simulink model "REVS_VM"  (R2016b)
settings: Solver=ode3  StartTime=REVS.sim_start_time_secs  StopTime=Inf  FixedStep=REVS.sim_step_time_secs  MaxStep=REVS.sim_step_time_secs  EnableMultiTasking=on
StopFcn:
  | postproc_datalog;
  | postproc_audit;
  | postproc_result;
model workspace (MATLAB code in the model file):
  other statements: REVS_setup_variants
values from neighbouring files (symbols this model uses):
  accessory = class_accessory_data    [class_test_data.m]
  battery = class_battery_data    [class_accessory_data.m]    (also in class_REVS_electric.m = class_REVS_battery)
  brake = struct(	'max_torque_Nm',[], 						'proportion_norm',1.0, 						'inertia_kgm2',0.0)    [class_REVS_drive_axle.m]
  engine = class_engine_data    [class_test_data.m]
  final_drive = struct(	'gear_ratio',[], 								'efficiency_norm',[], 								'inertia_kgm2',[] )    [class_REVS_drive_axle.m]
  gear = class_REVS_gearbox    [class_REVS_AT_transmission.m]
  tire = struct(	'radius_m',[], 						'rolling_resistance_coefficient',0, 						'vehicle_weight_norm',1.0,  						'wheel_slip_torque_Nm',[],  						'inertia_kgm2',0.0)    [class_REVS_drive_axle.m]
  torque_converter = class_REVS_torque_converter    [class_REVS_AT_transmission.m]
  transmission = class_transmission_data    [class_test_data.m]
  vehicle = class_vehicle_data    [class_test_data.m]
undefined symbols (not defined in the file or in its folder): alternator, ambient, controls, convert, DelayTimeSecs, drive_cycle, driver, electric, gear_strategy, InitialCondition, InitialValue, LoadSource, LookupStructure, MultiplyPosInputs, Normalize, NumPhases, REVS, SpeedSource, starter, tableshift, UpperSaturationLimit, Value, VerboseLevel, VerboseSignal
libraries: simulink x153
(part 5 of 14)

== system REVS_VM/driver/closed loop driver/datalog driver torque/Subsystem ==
  In1 : Inport
  Enable : EnablePort
  To Workspace : ToWorkspace  VariableName=datalog__driver__p_pedal_unscaled  SampleTime=-1
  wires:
  In1/1 -> To Workspace/1

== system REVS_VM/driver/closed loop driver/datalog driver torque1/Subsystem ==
  In1 : Inport
  Enable : EnablePort
  To Workspace : ToWorkspace  VariableName=datalog__driver__i_pedal_unscaled  SampleTime=-1
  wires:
  In1/1 -> To Workspace/1

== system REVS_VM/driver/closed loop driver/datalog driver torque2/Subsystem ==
  In1 : Inport
  Enable : EnablePort
  To Workspace : ToWorkspace  VariableName=datalog__driver__d_pedal_unscaled  SampleTime=-1
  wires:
  In1/1 -> To Workspace/1

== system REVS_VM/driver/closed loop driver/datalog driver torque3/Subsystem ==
  In1 : Inport
  Enable : EnablePort
  To Workspace : ToWorkspace  VariableName=datalog__driver__driveline_enagaged_bool  SampleTime=-1
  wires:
  In1/1 -> To Workspace/1

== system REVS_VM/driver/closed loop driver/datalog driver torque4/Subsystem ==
  In1 : Inport
  Enable : EnablePort
  To Workspace : ToWorkspace  VariableName=datalog__driver__driveline_enagaged_norm  SampleTime=-1
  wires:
  In1/1 -> To Workspace/1

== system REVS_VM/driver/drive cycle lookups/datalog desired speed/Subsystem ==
  In1 : Inport
  Enable : EnablePort
  To Workspace : ToWorkspace  VariableName=datalog__drive_cycle_speed_mps  SampleTime=-1
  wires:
  In1/1 -> To Workspace/1

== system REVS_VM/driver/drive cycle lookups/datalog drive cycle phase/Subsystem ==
  In1 : Inport
  Enable : EnablePort
  To Workspace : ToWorkspace  VariableName=datalog__drive_cycle_phase  SampleTime=-1
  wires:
  In1/1 -> To Workspace/1

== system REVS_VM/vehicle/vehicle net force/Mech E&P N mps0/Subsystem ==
  force_N : Inport
  spd_mps : Inport  Port=2
  Enable : EnablePort  ZeroCross=off
  Integrator1 : Integrator  LimitOutput=on  UpperSaturationLimit=Inf  LowerSaturationLimit=0  ZeroCross=off
  Mech Energy N mps : Subsystem  TreatAsAtomicUnit=on
  distance_to_workspace : ToWorkspace  VariableName=audit__mech__vehicle__gradient_drag_m  SampleTime=-1
  energy_to_workspace : ToWorkspace  VariableName=audit__mech__vehicle__gradient_drag_kJ  SampleTime=-1
  force_to_workspace : ToWorkspace  VariableName=audit__mech__vehicle__gradient_drag_N  SampleTime=-1
  neg_energy_to_workspace : ToWorkspace  VariableName=audit__mech__vehicle__gradient_drag_neg_kJ  SampleTime=-1
  pos_energy_to_workspace : ToWorkspace  VariableName=audit__mech__vehicle__gradient_drag_pos_kJ  SampleTime=-1
  power_to_workspace : ToWorkspace  VariableName=audit__mech__vehicle__gradient_drag_kW  SampleTime=-1
  speed_to_workspace : ToWorkspace  VariableName=audit__mech__vehicle__gradient_drag_mps  SampleTime=-1
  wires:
  Integrator1/1 -> distance_to_workspace/1
  spd_mps/1 -> Mech Energy N mps/2(spd_mps), speed_to_workspace/1, Integrator1/1
  force_N/1 -> Mech Energy N mps/1(force_N), force_to_workspace/1
  Mech Energy N mps/1("total_kJ ") -> energy_to_workspace/1
  Mech Energy N mps/4(pwr_kW) -> power_to_workspace/1
  Mech Energy N mps/2("pos_kJ ") -> pos_energy_to_workspace/1
  Mech Energy N mps/3(neg_kJ) -> neg_energy_to_workspace/1

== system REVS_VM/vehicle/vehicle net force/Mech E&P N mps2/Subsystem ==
  force_N : Inport
  spd_mps : Inport  Port=2
  Enable : EnablePort  ZeroCross=off
  Integrator1 : Integrator  LimitOutput=on  UpperSaturationLimit=Inf  LowerSaturationLimit=0  ZeroCross=off
  Mech Energy N mps : Subsystem  TreatAsAtomicUnit=on
  distance_to_workspace : ToWorkspace  VariableName=audit__mech__vehicle__ABC_drag_m  SampleTime=-1
  energy_to_workspace : ToWorkspace  VariableName=audit__mech__vehicle__ABC_drag_kJ  SampleTime=-1
  force_to_workspace : ToWorkspace  VariableName=audit__mech__vehicle__ABC_drag_N  SampleTime=-1
  neg_energy_to_workspace : ToWorkspace  VariableName=audit__mech__vehicle__ABC_drag_neg_kJ  SampleTime=-1
  pos_energy_to_workspace : ToWorkspace  VariableName=audit__mech__vehicle__ABC_drag_pos_kJ  SampleTime=-1
  power_to_workspace : ToWorkspace  VariableName=audit__mech__vehicle__ABC_drag_kW  SampleTime=-1
  speed_to_workspace : ToWorkspace  VariableName=audit__mech__vehicle__ABC_drag_mps  SampleTime=-1
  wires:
  Integrator1/1 -> distance_to_workspace/1
  spd_mps/1 -> Mech Energy N mps/2(spd_mps), speed_to_workspace/1, Integrator1/1
  force_N/1 -> Mech Energy N mps/1(force_N), force_to_workspace/1
  Mech Energy N mps/1("total_kJ ") -> energy_to_workspace/1
  Mech Energy N mps/4(pwr_kW) -> power_to_workspace/1
  Mech Energy N mps/2("pos_kJ ") -> pos_energy_to_workspace/1
  Mech Energy N mps/3(neg_kJ) -> neg_energy_to_workspace/1

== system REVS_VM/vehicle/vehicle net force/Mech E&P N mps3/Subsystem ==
  force_N : Inport
  spd_mps : Inport  Port=2
  mass_kg : Inport  Port=3
  Enable : EnablePort  ZeroCross=off
  Integrator1 : Integrator  LimitOutput=on  UpperSaturationLimit=Inf  LowerSaturationLimit=0  ZeroCross=off
  KE_to_workspace : ToWorkspace  VariableName=audit__mech__vehicle__input_KE_kJ  SampleTime=-1
  Mech Energy N mps : Subsystem  TreatAsAtomicUnit=on
  Mult : Product  Inputs=**
  Square : Math  Operator=square
  distance_to_workspace : ToWorkspace  VariableName=audit__mech__vehicle__input_m  SampleTime=-1
  energy_to_workspace : ToWorkspace  VariableName=audit__mech__vehicle__input_kJ  SampleTime=-1
  force_to_workspace : ToWorkspace  VariableName=audit__mech__vehicle__input_N  SampleTime=-1
  mass_to_workspace : ToWorkspace  VariableName=audit__mech__vehicle__input_kg  SampleTime=-1
  neg_energy_to_workspace : ToWorkspace  VariableName=audit__mech__vehicle__input_neg_kJ  SampleTime=-1
  one half : Gain  Gain=0.5/1000
  pos_energy_to_workspace : ToWorkspace  VariableName=audit__mech__vehicle__input_pos_kJ  SampleTime=-1
  power_to_workspace : ToWorkspace  VariableName=audit__mech__vehicle__input_kW  SampleTime=-1
  speed_to_workspace : ToWorkspace  VariableName=audit__mech__vehicle__input_mps  SampleTime=-1
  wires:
  Integrator1/1 -> distance_to_workspace/1
  force_N/1 -> force_to_workspace/1, Mech Energy N mps/1(force_N)
  spd_mps/1 -> speed_to_workspace/1, Square/1, Integrator1/1, Mech Energy N mps/2(spd_mps)
  mass_kg/1 -> mass_to_workspace/1, Mult/2
  Mult/1 -> one half/1
  Square/1 -> Mult/1
  one half/1 -> KE_to_workspace/1
  Mech Energy N mps/3(neg_kJ) -> neg_energy_to_workspace/1
  Mech Energy N mps/2("pos_kJ ") -> pos_energy_to_workspace/1
  Mech Energy N mps/4(pwr_kW) -> power_to_workspace/1
  Mech Energy N mps/1("total_kJ ") -> energy_to_workspace/1

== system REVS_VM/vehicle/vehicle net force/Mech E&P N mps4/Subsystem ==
  force_N : Inport
  spd_mps : Inport  Port=2
  Enable : EnablePort  ZeroCross=off
  Integrator1 : Integrator  LimitOutput=on  UpperSaturationLimit=Inf  LowerSaturationLimit=0  ZeroCross=off
  Mech Energy N mps : Subsystem  TreatAsAtomicUnit=on
  distance_to_workspace : ToWorkspace  VariableName=audit__mech__vehicle__aerodynamic_drag_m  SampleTime=-1
  energy_to_workspace : ToWorkspace  VariableName=audit__mech__vehicle__aerodynamic_drag_kJ  SampleTime=-1
  force_to_workspace : ToWorkspace  VariableName=audit__mech__vehicle__aerodynamic_drag_N  SampleTime=-1
  neg_energy_to_workspace : ToWorkspace  VariableName=audit__mech__vehicle__aerodynamic_drag_neg_kJ  SampleTime=-1
  pos_energy_to_workspace : ToWorkspace  VariableName=audit__mech__vehicle__aerodynamic_drag_pos_kJ  SampleTime=-1
  power_to_workspace : ToWorkspace  VariableName=audit__mech__vehicle__aerodynamic_drag_kW  SampleTime=-1
  speed_to_workspace : ToWorkspace  VariableName=audit__mech__vehicle__aerodynamic_drag_mps  SampleTime=-1
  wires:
  Integrator1/1 -> distance_to_workspace/1
  spd_mps/1 -> Mech Energy N mps/2(spd_mps), speed_to_workspace/1, Integrator1/1
  force_N/1 -> Mech Energy N mps/1(force_N), force_to_workspace/1
  Mech Energy N mps/1("total_kJ ") -> energy_to_workspace/1
  Mech Energy N mps/4(pwr_kW) -> power_to_workspace/1
  Mech Energy N mps/2("pos_kJ ") -> pos_energy_to_workspace/1
  Mech Energy N mps/3(neg_kJ) -> neg_energy_to_workspace/1

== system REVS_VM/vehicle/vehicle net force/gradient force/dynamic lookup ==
  bus : Inport
  Bus Selector : BusSelector  OutputSignals=gb.gb_cmd_gear,gb_spd_in_radps,ctrl.gb_line_press_bar
  Lookup : Lookup_n-D  NumberOfTableDimensions=10  BreakpointsForDimension1=LookupStructure.axis_1.breakpoints  BreakpointsForDimension2=LookupStructure.axis_2.breakpoints  BreakpointsForDimension3=LookupStructure.axis_3.breakpoints  BreakpointsForDimension4=LookupStructure.axis_4.breakpoints  BreakpointsForDimension5=LookupStructure.axis_5.breakpoints  BreakpointsForDimension6=LookupStructure.axis_6.breakpoints  BreakpointsForDimension7=LookupStructure.axis_7.breakpoints  BreakpointsForDimension8=LookupStructure.axis_8.breakpoints  BreakpointsForDimension9=LookupStructure.axis_9.breakpoints  BreakpointsForDimension10=LookupStructure.axis_10.breakpoints  IndexSearchMethod=Linear search  BeginIndexSearchUsingPreviousIndexResult=on  Table=LookupStructure.table  DiagnosticForOutOfRangeInput=Warning  InternalRulePriority=Speed  RndMeth=Simplest  SupportTunableTableSize=on  MaximumIndicesForEachDimension=LookupStructure.table_size
  out : Outport
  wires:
  bus/1 -> Bus Selector/1
  Lookup/1 -> out/1

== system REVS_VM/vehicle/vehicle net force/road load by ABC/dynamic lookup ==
  bus : Inport
  Bus Selector : BusSelector  OutputSignals=gb.gb_cmd_gear,gb_spd_in_radps,ctrl.gb_line_press_bar
  Lookup : Lookup_n-D  NumberOfTableDimensions=10  BreakpointsForDimension1=LookupStructure.axis_1.breakpoints  BreakpointsForDimension2=LookupStructure.axis_2.breakpoints  BreakpointsForDimension3=LookupStructure.axis_3.breakpoints  BreakpointsForDimension4=LookupStructure.axis_4.breakpoints  BreakpointsForDimension5=LookupStructure.axis_5.breakpoints  BreakpointsForDimension6=LookupStructure.axis_6.breakpoints  BreakpointsForDimension7=LookupStructure.axis_7.breakpoints  BreakpointsForDimension8=LookupStructure.axis_8.breakpoints  BreakpointsForDimension9=LookupStructure.axis_9.breakpoints  BreakpointsForDimension10=LookupStructure.axis_10.breakpoints  IndexSearchMethod=Linear search  BeginIndexSearchUsingPreviousIndexResult=on  Table=LookupStructure.table  DiagnosticForOutOfRangeInput=Warning  InternalRulePriority=Speed  RndMeth=Simplest  SupportTunableTableSize=on  MaximumIndicesForEachDimension=LookupStructure.table_size
  out : Outport
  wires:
  bus/1 -> Bus Selector/1
  Lookup/1 -> out/1

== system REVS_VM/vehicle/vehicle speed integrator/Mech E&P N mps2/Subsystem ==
  force_N : Inport
  spd_mps : Inport  Port=2
  mass_kg : Inport  Port=3
  Enable : EnablePort  ZeroCross=off
  Integrator1 : Integrator  LimitOutput=on  UpperSaturationLimit=Inf  LowerSaturationLimit=0  ZeroCross=off
  KE_to_workspace : ToWorkspace  VariableName=audit__mech__vehicle__output_KE_kJ  SampleTime=-1
  Mech Energy N mps : Subsystem  TreatAsAtomicUnit=on
  Mult : Product  Inputs=**
  Square : Math  Operator=square
  distance_to_workspace : ToWorkspace  VariableName=audit__mech__vehicle__output_m  SampleTime=-1
  energy_to_workspace : ToWorkspace  VariableName=audit__mech__vehicle__output_kJ  SampleTime=-1
  force_to_workspace : ToWorkspace  VariableName=audit__mech__vehicle__output_N  SampleTime=-1
  mass_to_workspace : ToWorkspace  VariableName=audit__mech__vehicle__output_kg  SampleTime=-1
  neg_energy_to_workspace : ToWorkspace  VariableName=audit__mech__vehicle__output_neg_kJ  SampleTime=-1
  one half : Gain  Gain=0.5/1000
  pos_energy_to_workspace : ToWorkspace  VariableName=audit__mech__vehicle__output_pos_kJ  SampleTime=-1
  power_to_workspace : ToWorkspace  VariableName=audit__mech__vehicle__output_kW  SampleTime=-1
  speed_to_workspace : ToWorkspace  VariableName=audit__mech__vehicle__output_mps  SampleTime=-1
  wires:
  Integrator1/1 -> distance_to_workspace/1
  force_N/1 -> force_to_workspace/1, Mech Energy N mps/1(force_N)
  spd_mps/1 -> speed_to_workspace/1, Square/1, Integrator1/1, Mech Energy N mps/2(spd_mps)
  mass_kg/1 -> mass_to_workspace/1, Mult/2
  Mult/1 -> one half/1
  Square/1 -> Mult/1
  one half/1 -> KE_to_workspace/1
  Mech Energy N mps/3(neg_kJ) -> neg_energy_to_workspace/1
  Mech Energy N mps/2("pos_kJ ") -> pos_energy_to_workspace/1
  Mech Energy N mps/4(pwr_kW) -> power_to_workspace/1
  Mech Energy N mps/1("total_kJ ") -> energy_to_workspace/1

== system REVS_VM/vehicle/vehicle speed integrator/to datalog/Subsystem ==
  In1 : Inport
  Enable : EnablePort
  To Workspace : ToWorkspace  VariableName=datalog__vehicle__dynamic_mass_kg  SampleTime=-1
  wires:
  In1/1 -> To Workspace/1

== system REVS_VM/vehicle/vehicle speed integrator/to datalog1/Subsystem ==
  In1 : Inport
  Enable : EnablePort
  To Workspace : ToWorkspace  VariableName=datalog__vehicle__speed_mps  SampleTime=-1
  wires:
  In1/1 -> To Workspace/1

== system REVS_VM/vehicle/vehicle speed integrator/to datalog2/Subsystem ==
  In1 : Inport
  Enable : EnablePort
  To Workspace : ToWorkspace  VariableName=datalog__vehicle__distance_m  SampleTime=-1
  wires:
  In1/1 -> To Workspace/1

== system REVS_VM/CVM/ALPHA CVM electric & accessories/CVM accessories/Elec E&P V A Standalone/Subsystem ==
  volts_V : Inport
  curr_A : Inport  Port=2
  Enable : EnablePort  ZeroCross=off
  Elec Energy V A : Subsystem  TreatAsAtomicUnit=on
  amps_to_workspace : ToWorkspace  VariableName=audit__elec__accessories__total_Amps  SampleTime=-1
  energy_to_workspace : ToWorkspace  VariableName=audit__elec__accessories__total_kJ  SampleTime=-1
  neg_energy_to_workspace : ToWorkspace  VariableName=audit__elec__accessories__total_neg_kJ  SampleTime=-1
  pos_energy_to_workspace : ToWorkspace  VariableName=audit__elec__accessories__total_pos_kJ  SampleTime=-1
  power_to_workspace : ToWorkspace  VariableName=audit__elec__accessories__total_kW  SampleTime=-1
  volts_to_workspace : ToWorkspace  VariableName=audit__elec__accessories__total_Volts  SampleTime=-1
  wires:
  Elec Energy V A/1("total_kJ ") -> energy_to_workspace/1
  Elec Energy V A/4(pwr_kW) -> power_to_workspace/1
  Elec Energy V A/2("pos_kJ ") -> pos_energy_to_workspace/1
  Elec Energy V A/3(neg_kJ) -> neg_energy_to_workspace/1
  curr_A/1 -> amps_to_workspace/1, Elec Energy V A/2(curr_A)
  volts_V/1 -> volts_to_workspace/1, Elec Energy V A/1(volts_V)

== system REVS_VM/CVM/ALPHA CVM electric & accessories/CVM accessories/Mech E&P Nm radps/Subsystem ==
  trq_Nm : Inport
  spd_radps : Inport  Port=2
  Enable : EnablePort  ZeroCross=off
  Mech Energy Nm radps : Subsystem  TreatAsAtomicUnit=on
  energy_to_workspace : ToWorkspace  VariableName=audit__mech__accessories__total_kJ  SampleTime=-1
  neg_energy_to_workspace : ToWorkspace  VariableName=audit__mech__accessories__total_neg_kJ  SampleTime=-1
  pos_energy_to_workspace : ToWorkspace  VariableName=audit__mech__accessories__total_pos_kJ  SampleTime=-1
  power_to_workspace : ToWorkspace  VariableName=audit__mech__accessories__total_kW  SampleTime=-1
  speed_to_workspace : ToWorkspace  VariableName=audit__mech__accessories__total_radps  SampleTime=-1
  torque_to_workspace : ToWorkspace  VariableName=audit__mech__accessories__total_Nm  SampleTime=-1
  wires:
  spd_radps/1 -> Mech Energy Nm radps/2(spd_radps), speed_to_workspace/1
  trq_Nm/1 -> Mech Energy Nm radps/1(trq_Nm), torque_to_workspace/1
  Mech Energy Nm radps/3(neg_kJ) -> neg_energy_to_workspace/1
  Mech Energy Nm radps/2("pos_kJ ") -> pos_energy_to_workspace/1
  Mech Energy Nm radps/4(pwr_kW) -> power_to_workspace/1
  Mech Energy Nm radps/1("total_kJ ") -> energy_to_workspace/1

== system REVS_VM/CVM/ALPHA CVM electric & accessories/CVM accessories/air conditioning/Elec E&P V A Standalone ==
  volts_V : Inport
  curr_A : Inport  Port=2
  Compare To Constant : simulink/Logic and Bit Operations/Compare To Constant  relop=>=  const=1  OutDataTypeStr=boolean
  Constant : Constant  Value=VerboseSignal
  Subsystem : Subsystem
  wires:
  volts_V/1 -> Subsystem/1(volts_V)
  curr_A/1 -> Subsystem/2(curr_A)
  Compare To Constant/1 -> Subsystem/Enable
  Constant/1 -> Compare To Constant/1

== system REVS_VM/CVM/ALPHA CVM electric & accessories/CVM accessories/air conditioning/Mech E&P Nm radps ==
  " trq_Nm" : Inport
  spd_radps : Inport  Port=2
  iner_kgm2 : Inport  Port=3
  Compare To Constant : simulink/Logic and Bit Operations/Compare To Constant  relop=>=  const=1  OutDataTypeStr=boolean
  Constant : Constant  Value=VerboseSignal
  Subsystem : Subsystem
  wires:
  " trq_Nm"/1 -> Subsystem/1(" trq_Nm")
  spd_radps/1 -> Subsystem/2(spd_radps)
  iner_kgm2/1 -> Subsystem/3(iner_kgm2)
  Compare To Constant/1 -> Subsystem/Enable
  Constant/1 -> Compare To Constant/1

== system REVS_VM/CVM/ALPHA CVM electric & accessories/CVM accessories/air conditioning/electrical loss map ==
  bus : Inport
  Bus Selector : BusSelector  OutputSignals=gb.gb_cmd_gear,gb_spd_in_radps,ctrl.gb_line_press_bar
  Lookup : Lookup_n-D  NumberOfTableDimensions=10  BreakpointsForDimension1=LookupStructure.axis_1.breakpoints  BreakpointsForDimension2=LookupStructure.axis_2.breakpoints  BreakpointsForDimension3=LookupStructure.axis_3.breakpoints  BreakpointsForDimension4=LookupStructure.axis_4.breakpoints  BreakpointsForDimension5=LookupStructure.axis_5.breakpoints  BreakpointsForDimension6=LookupStructure.axis_6.breakpoints  BreakpointsForDimension7=LookupStructure.axis_7.breakpoints  BreakpointsForDimension8=LookupStructure.axis_8.breakpoints  BreakpointsForDimension9=LookupStructure.axis_9.breakpoints  BreakpointsForDimension10=LookupStructure.axis_10.breakpoints  IndexSearchMethod=Linear search  BeginIndexSearchUsingPreviousIndexResult=on  Table=LookupStructure.table  DiagnosticForOutOfRangeInput=Warning  InternalRulePriority=Speed  RndMeth=Simplest  SupportTunableTableSize=on  MaximumIndicesForEachDimension=LookupStructure.table_size
  out : Outport
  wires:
  bus/1 -> Bus Selector/1
  Lookup/1 -> out/1

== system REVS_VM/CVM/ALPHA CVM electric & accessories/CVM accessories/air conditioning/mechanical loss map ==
  bus : Inport
  Bus Selector : BusSelector  OutputSignals=gb.gb_cmd_gear,gb_spd_in_radps,ctrl.gb_line_press_bar
  Lookup : Lookup_n-D  NumberOfTableDimensions=10  BreakpointsForDimension1=LookupStructure.axis_1.breakpoints  BreakpointsForDimension2=LookupStructure.axis_2.breakpoints  BreakpointsForDimension3=LookupStructure.axis_3.breakpoints  BreakpointsForDimension4=LookupStructure.axis_4.breakpoints  BreakpointsForDimension5=LookupStructure.axis_5.breakpoints  BreakpointsForDimension6=LookupStructure.axis_6.breakpoints  BreakpointsForDimension7=LookupStructure.axis_7.breakpoints  BreakpointsForDimension8=LookupStructure.axis_8.breakpoints  BreakpointsForDimension9=LookupStructure.axis_9.breakpoints  BreakpointsForDimension10=LookupStructure.axis_10.breakpoints  IndexSearchMethod=Linear search  BeginIndexSearchUsingPreviousIndexResult=on  Table=LookupStructure.table  DiagnosticForOutOfRangeInput=Warning  InternalRulePriority=Speed  RndMeth=Simplest  SupportTunableTableSize=on  MaximumIndicesForEachDimension=LookupStructure.table_size
  out : Outport
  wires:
  bus/1 -> Bus Selector/1
  Lookup/1 -> out/1

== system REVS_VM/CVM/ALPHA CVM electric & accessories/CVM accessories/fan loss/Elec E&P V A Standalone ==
  volts_V : Inport
  curr_A : Inport  Port=2
  Compare To Constant : simulink/Logic and Bit Operations/Compare To Constant  relop=>=  const=1  OutDataTypeStr=boolean
  Constant : Constant  Value=VerboseSignal
  Subsystem : Subsystem
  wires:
  volts_V/1 -> Subsystem/1(volts_V)
  curr_A/1 -> Subsystem/2(curr_A)
  Compare To Constant/1 -> Subsystem/Enable
  Constant/1 -> Compare To Constant/1

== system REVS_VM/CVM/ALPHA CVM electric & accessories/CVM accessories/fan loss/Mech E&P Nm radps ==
  " trq_Nm" : Inport
  spd_radps : Inport  Port=2
  iner_kgm2 : Inport  Port=3
  Compare To Constant : simulink/Logic and Bit Operations/Compare To Constant  relop=>=  const=1  OutDataTypeStr=boolean
  Constant : Constant  Value=VerboseSignal
  Subsystem : Subsystem
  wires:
  " trq_Nm"/1 -> Subsystem/1(" trq_Nm")
  spd_radps/1 -> Subsystem/2(spd_radps)
  iner_kgm2/1 -> Subsystem/3(iner_kgm2)
  Compare To Constant/1 -> Subsystem/Enable
  Constant/1 -> Compare To Constant/1

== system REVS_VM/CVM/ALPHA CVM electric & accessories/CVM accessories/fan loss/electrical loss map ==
  bus : Inport
  Bus Selector : BusSelector  OutputSignals=gb.gb_cmd_gear,gb_spd_in_radps,ctrl.gb_line_press_bar
  Lookup : Lookup_n-D  NumberOfTableDimensions=10  BreakpointsForDimension1=LookupStructure.axis_1.breakpoints  BreakpointsForDimension2=LookupStructure.axis_2.breakpoints  BreakpointsForDimension3=LookupStructure.axis_3.breakpoints  BreakpointsForDimension4=LookupStructure.axis_4.breakpoints  BreakpointsForDimension5=LookupStructure.axis_5.breakpoints  BreakpointsForDimension6=LookupStructure.axis_6.breakpoints  BreakpointsForDimension7=LookupStructure.axis_7.breakpoints  BreakpointsForDimension8=LookupStructure.axis_8.breakpoints  BreakpointsForDimension9=LookupStructure.axis_9.breakpoints  BreakpointsForDimension10=LookupStructure.axis_10.breakpoints  IndexSearchMethod=Linear search  BeginIndexSearchUsingPreviousIndexResult=on  Table=LookupStructure.table  DiagnosticForOutOfRangeInput=Warning  InternalRulePriority=Speed  RndMeth=Simplest  SupportTunableTableSize=on  MaximumIndicesForEachDimension=LookupStructure.table_size
  out : Outport
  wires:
  bus/1 -> Bus Selector/1
  Lookup/1 -> out/1

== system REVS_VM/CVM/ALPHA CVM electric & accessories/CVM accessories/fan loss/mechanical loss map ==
  bus : Inport
  Bus Selector : BusSelector  OutputSignals=gb.gb_cmd_gear,gb_spd_in_radps,ctrl.gb_line_press_bar
  Lookup : Lookup_n-D  NumberOfTableDimensions=10  BreakpointsForDimension1=LookupStructure.axis_1.breakpoints  BreakpointsForDimension2=LookupStructure.axis_2.breakpoints  BreakpointsForDimension3=LookupStructure.axis_3.breakpoints  BreakpointsForDimension4=LookupStructure.axis_4.breakpoints  BreakpointsForDimension5=LookupStructure.axis_5.breakpoints  BreakpointsForDimension6=LookupStructure.axis_6.breakpoints  BreakpointsForDimension7=LookupStructure.axis_7.breakpoints  BreakpointsForDimension8=LookupStructure.axis_8.breakpoints  BreakpointsForDimension9=LookupStructure.axis_9.breakpoints  BreakpointsForDimension10=LookupStructure.axis_10.breakpoints  IndexSearchMethod=Linear search  BeginIndexSearchUsingPreviousIndexResult=on  Table=LookupStructure.table  DiagnosticForOutOfRangeInput=Warning  InternalRulePriority=Speed  RndMeth=Simplest  SupportTunableTableSize=on  MaximumIndicesForEachDimension=LookupStructure.table_size
  out : Outport
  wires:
  bus/1 -> Bus Selector/1
  Lookup/1 -> out/1

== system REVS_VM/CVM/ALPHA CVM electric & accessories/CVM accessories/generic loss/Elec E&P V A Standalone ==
  volts_V : Inport
  curr_A : Inport  Port=2
  Compare To Constant : simulink/Logic and Bit Operations/Compare To Constant  relop=>=  const=1  OutDataTypeStr=boolean
  Constant : Constant  Value=VerboseSignal
  Subsystem : Subsystem
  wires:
  volts_V/1 -> Subsystem/1(volts_V)
  curr_A/1 -> Subsystem/2(curr_A)
  Compare To Constant/1 -> Subsystem/Enable
  Constant/1 -> Compare To Constant/1

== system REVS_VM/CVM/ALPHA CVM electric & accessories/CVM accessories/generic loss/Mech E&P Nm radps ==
  " trq_Nm" : Inport
  spd_radps : Inport  Port=2
  iner_kgm2 : Inport  Port=3
  Compare To Constant : simulink/Logic and Bit Operations/Compare To Constant  relop=>=  const=1  OutDataTypeStr=boolean
  Constant : Constant  Value=VerboseSignal
  Subsystem : Subsystem
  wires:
  " trq_Nm"/1 -> Subsystem/1(" trq_Nm")
  spd_radps/1 -> Subsystem/2(spd_radps)
  iner_kgm2/1 -> Subsystem/3(iner_kgm2)
  Compare To Constant/1 -> Subsystem/Enable
  Constant/1 -> Compare To Constant/1

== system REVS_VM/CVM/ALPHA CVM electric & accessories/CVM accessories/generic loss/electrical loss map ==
  bus : Inport
  Bus Selector : BusSelector  OutputSignals=gb.gb_cmd_gear,gb_spd_in_radps,ctrl.gb_line_press_bar
  Lookup : Lookup_n-D  NumberOfTableDimensions=10  BreakpointsForDimension1=LookupStructure.axis_1.breakpoints  BreakpointsForDimension2=LookupStructure.axis_2.breakpoints  BreakpointsForDimension3=LookupStructure.axis_3.breakpoints  BreakpointsForDimension4=LookupStructure.axis_4.breakpoints  BreakpointsForDimension5=LookupStructure.axis_5.breakpoints  BreakpointsForDimension6=LookupStructure.axis_6.breakpoints  BreakpointsForDimension7=LookupStructure.axis_7.breakpoints  BreakpointsForDimension8=LookupStructure.axis_8.breakpoints  BreakpointsForDimension9=LookupStructure.axis_9.breakpoints  BreakpointsForDimension10=LookupStructure.axis_10.breakpoints  IndexSearchMethod=Linear search  BeginIndexSearchUsingPreviousIndexResult=on  Table=LookupStructure.table  DiagnosticForOutOfRangeInput=Warning  InternalRulePriority=Speed  RndMeth=Simplest  SupportTunableTableSize=on  MaximumIndicesForEachDimension=LookupStructure.table_size
  out : Outport
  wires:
  bus/1 -> Bus Selector/1
  Lookup/1 -> out/1

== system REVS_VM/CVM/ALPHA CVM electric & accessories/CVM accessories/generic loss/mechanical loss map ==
  bus : Inport
  Bus Selector : BusSelector  OutputSignals=gb.gb_cmd_gear,gb_spd_in_radps,ctrl.gb_line_press_bar
  Lookup : Lookup_n-D  NumberOfTableDimensions=10  BreakpointsForDimension1=LookupStructure.axis_1.breakpoints  BreakpointsForDimension2=LookupStructure.axis_2.breakpoints  BreakpointsForDimension3=LookupStructure.axis_3.breakpoints  BreakpointsForDimension4=LookupStructure.axis_4.breakpoints  BreakpointsForDimension5=LookupStructure.axis_5.breakpoints  BreakpointsForDimension6=LookupStructure.axis_6.breakpoints  BreakpointsForDimension7=LookupStructure.axis_7.breakpoints  BreakpointsForDimension8=LookupStructure.axis_8.breakpoints  BreakpointsForDimension9=LookupStructure.axis_9.breakpoints  BreakpointsForDimension10=LookupStructure.axis_10.breakpoints  IndexSearchMethod=Linear search  BeginIndexSearchUsingPreviousIndexResult=on  Table=LookupStructure.table  DiagnosticForOutOfRangeInput=Warning  InternalRulePriority=Speed  RndMeth=Simplest  SupportTunableTableSize=on  MaximumIndicesForEachDimension=LookupStructure.table_size
  out : Outport
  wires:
  bus/1 -> Bus Selector/1
  Lookup/1 -> out/1

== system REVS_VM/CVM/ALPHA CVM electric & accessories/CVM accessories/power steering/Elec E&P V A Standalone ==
  volts_V : Inport
  curr_A : Inport  Port=2
  Compare To Constant : simulink/Logic and Bit Operations/Compare To Constant  relop=>=  const=1  OutDataTypeStr=boolean
  Constant : Constant  Value=VerboseSignal
  Subsystem : Subsystem
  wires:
  volts_V/1 -> Subsystem/1(volts_V)
  curr_A/1 -> Subsystem/2(curr_A)
  Compare To Constant/1 -> Subsystem/Enable
  Constant/1 -> Compare To Constant/1

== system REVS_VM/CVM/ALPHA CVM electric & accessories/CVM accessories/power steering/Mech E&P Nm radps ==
  " trq_Nm" : Inport
  spd_radps : Inport  Port=2
  iner_kgm2 : Inport  Port=3
  Compare To Constant : simulink/Logic and Bit Operations/Compare To Constant  relop=>=  const=1  OutDataTypeStr=boolean
  Constant : Constant  Value=VerboseSignal
  Subsystem : Subsystem
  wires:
  " trq_Nm"/1 -> Subsystem/1(" trq_Nm")
  spd_radps/1 -> Subsystem/2(spd_radps)
  iner_kgm2/1 -> Subsystem/3(iner_kgm2)
  Compare To Constant/1 -> Subsystem/Enable
  Constant/1 -> Compare To Constant/1

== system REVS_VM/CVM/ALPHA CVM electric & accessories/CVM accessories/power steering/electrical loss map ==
  bus : Inport
  Bus Selector : BusSelector  OutputSignals=gb.gb_cmd_gear,gb_spd_in_radps,ctrl.gb_line_press_bar
  Lookup : Lookup_n-D  NumberOfTableDimensions=10  BreakpointsForDimension1=LookupStructure.axis_1.breakpoints  BreakpointsForDimension2=LookupStructure.axis_2.breakpoints  BreakpointsForDimension3=LookupStructure.axis_3.breakpoints  BreakpointsForDimension4=LookupStructure.axis_4.breakpoints  BreakpointsForDimension5=LookupStructure.axis_5.breakpoints  BreakpointsForDimension6=LookupStructure.axis_6.breakpoints  BreakpointsForDimension7=LookupStructure.axis_7.breakpoints  BreakpointsForDimension8=LookupStructure.axis_8.breakpoints  BreakpointsForDimension9=LookupStructure.axis_9.breakpoints  BreakpointsForDimension10=LookupStructure.axis_10.breakpoints  IndexSearchMethod=Linear search  BeginIndexSearchUsingPreviousIndexResult=on  Table=LookupStructure.table  DiagnosticForOutOfRangeInput=Warning  InternalRulePriority=Speed  RndMeth=Simplest  SupportTunableTableSize=on  MaximumIndicesForEachDimension=LookupStructure.table_size
  out : Outport
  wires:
  bus/1 -> Bus Selector/1
  Lookup/1 -> out/1

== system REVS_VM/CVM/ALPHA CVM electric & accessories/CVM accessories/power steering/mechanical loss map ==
  bus : Inport
  Bus Selector : BusSelector  OutputSignals=gb.gb_cmd_gear,gb_spd_in_radps,ctrl.gb_line_press_bar
  Lookup : Lookup_n-D  NumberOfTableDimensions=10  BreakpointsForDimension1=LookupStructure.axis_1.breakpoints  BreakpointsForDimension2=LookupStructure.axis_2.breakpoints  BreakpointsForDimension3=LookupStructure.axis_3.breakpoints  BreakpointsForDimension4=LookupStructure.axis_4.breakpoints  BreakpointsForDimension5=LookupStructure.axis_5.breakpoints  BreakpointsForDimension6=LookupStructure.axis_6.breakpoints  BreakpointsForDimension7=LookupStructure.axis_7.breakpoints  BreakpointsForDimension8=LookupStructure.axis_8.breakpoints  BreakpointsForDimension9=LookupStructure.axis_9.breakpoints  BreakpointsForDimension10=LookupStructure.axis_10.breakpoints  IndexSearchMethod=Linear search  BeginIndexSearchUsingPreviousIndexResult=on  Table=LookupStructure.table  DiagnosticForOutOfRangeInput=Warning  InternalRulePriority=Speed  RndMeth=Simplest  SupportTunableTableSize=on  MaximumIndicesForEachDimension=LookupStructure.table_size
  out : Outport
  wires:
  bus/1 -> Bus Selector/1
  Lookup/1 -> out/1

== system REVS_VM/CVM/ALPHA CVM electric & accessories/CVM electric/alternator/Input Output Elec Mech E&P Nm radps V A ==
  volts_in_V : Inport
  curr_in_A : Inport  Port=2
  trq_out_Nm : Inport  Port=3
  spd_out_radps : Inport  Port=4
  iner_out_kgm2 : Inport  Port=5
  Compare To Constant : simulink/Logic and Bit Operations/Compare To Constant  relop=>=  const=1  OutDataTypeStr=boolean
  Constant : Constant  Value=VerboseSignal
  Subsystem : Subsystem
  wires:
  volts_in_V/1 -> Subsystem/1(volts_in_V)
  curr_in_A/1 -> Subsystem/2(curr_in_A)
  trq_out_Nm/1 -> Subsystem/3(trq_out_Nm)
  spd_out_radps/1 -> Subsystem/4(spd_out_radps)
  iner_out_kgm2/1 -> Subsystem/5(iner_out_kgm2)
  Compare To Constant/1 -> Subsystem/Enable
  Constant/1 -> Compare To Constant/1

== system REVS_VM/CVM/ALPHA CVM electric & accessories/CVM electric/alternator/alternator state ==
  eng_on : Inport
  spd_in_radps : Inport  Port=2
  Compare To Zero : simulink/Logic and Bit Operations/Compare To Zero  relop===  OutDataTypeStr=boolean
  Compare To Zero1 : simulink/Logic and Bit Operations/Compare To Zero  relop=>  OutDataTypeStr=boolean
  Latch : Subsystem
  Logical Operator : Logic  AllPortsSameDT=off  OutDataTypeStr=boolean
  Logical Operator1 : Logic  Operator=OR  AllPortsSameDT=off  OutDataTypeStr=boolean
  Product : Product
  Relational Operator : RelationalOperator  Operator=>  OutDataTypeStr=boolean
  Relational Operator1 : RelationalOperator  Operator=<  OutDataTypeStr=boolean
  activation_speed_radps2 : Constant  Value=alternator.activate_speed_radps
  boolean integrator : Subsystem
  deactivation_speed_radps : Constant  Value=alternator.deactivate_speed_radps
  normalize : Gain  Gain=1/alternator.activation_time_secs
  state : Outport
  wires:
  normalize/1 -> Product/2
  eng_on/1 -> Logical Operator/1, Compare To Zero/1
  Compare To Zero1/1 -> Product/1
  boolean integrator/1(out) -> normalize/1
  Product/1 -> state/1
  Compare To Zero/1 -> Logical Operator1/2
  Relational Operator1/1 -> Logical Operator1/1
  Latch/1(State) -> boolean integrator/1(bool), Compare To Zero1/1
  deactivation_speed_radps/1 -> Relational Operator1/2
  Logical Operator/1 -> Latch/1(On)
  Logical Operator1/1 -> Latch/2(Off)
  activation_speed_radps2/1 -> Relational Operator/2
  spd_in_radps/1 -> Relational Operator1/1, Relational Operator/1
  Relational Operator/1 -> Logical Operator/2

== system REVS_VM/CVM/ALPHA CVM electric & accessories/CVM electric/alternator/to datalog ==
  Var : Inport
  Constant : Constant  Value=VerboseSignal
  Constant1 : Constant  Value=VerboseLevel
  Relational Operator : RelationalOperator  OutDataTypeStr=boolean  ZeroCross=off
  Subsystem : Subsystem
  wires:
  Constant1/1 -> Relational Operator/2
  Constant/1 -> Relational Operator/1
  Relational Operator/1 -> Subsystem/Enable
  Var/1 -> Subsystem/1(In1)

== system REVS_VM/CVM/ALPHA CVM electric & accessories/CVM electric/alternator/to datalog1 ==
  Var : Inport
  Constant : Constant  Value=VerboseSignal
  Constant1 : Constant  Value=VerboseLevel
  Relational Operator : RelationalOperator  OutDataTypeStr=boolean  ZeroCross=off
  Subsystem : Subsystem
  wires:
  Constant1/1 -> Relational Operator/2
  Constant/1 -> Relational Operator/1
  Relational Operator/1 -> Subsystem/Enable
  Var/1 -> Subsystem/1(In1)

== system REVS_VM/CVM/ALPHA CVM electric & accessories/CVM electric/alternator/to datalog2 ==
  Var : Inport
  Constant : Constant  Value=VerboseSignal
  Constant1 : Constant  Value=VerboseLevel
  Relational Operator : RelationalOperator  OutDataTypeStr=boolean  ZeroCross=off
  Subsystem : Subsystem
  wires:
  Constant1/1 -> Relational Operator/2
  Constant/1 -> Relational Operator/1
  Relational Operator/1 -> Subsystem/Enable
  Var/1 -> Subsystem/1(In1)

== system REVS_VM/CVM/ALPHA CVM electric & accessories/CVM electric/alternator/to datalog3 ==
  Var : Inport
  Constant : Constant  Value=VerboseSignal
  Constant1 : Constant  Value=VerboseLevel
  Relational Operator : RelationalOperator  OutDataTypeStr=boolean  ZeroCross=off
  Subsystem : Subsystem
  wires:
  Constant1/1 -> Relational Operator/2
  Constant/1 -> Relational Operator/1
  Relational Operator/1 -> Subsystem/Enable
  Var/1 -> Subsystem/1(In1)

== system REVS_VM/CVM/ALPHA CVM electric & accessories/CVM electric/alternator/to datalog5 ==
  Var : Inport
  Constant : Constant  Value=VerboseSignal
  Constant1 : Constant  Value=VerboseLevel
  Relational Operator : RelationalOperator  OutDataTypeStr=boolean  ZeroCross=off
  Subsystem : Subsystem
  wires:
  Constant1/1 -> Relational Operator/2
  Constant/1 -> Relational Operator/1
  Relational Operator/1 -> Subsystem/Enable
  Var/1 -> Subsystem/1(In1)

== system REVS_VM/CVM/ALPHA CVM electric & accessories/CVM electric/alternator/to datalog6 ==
  Var : Inport
  Constant : Constant  Value=VerboseSignal
  Constant1 : Constant  Value=VerboseLevel
  Relational Operator : RelationalOperator  OutDataTypeStr=boolean  ZeroCross=off
  Subsystem : Subsystem
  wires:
  Constant1/1 -> Relational Operator/2
  Constant/1 -> Relational Operator/1
  Relational Operator/1 -> Subsystem/Enable
  Var/1 -> Subsystem/1(In1)

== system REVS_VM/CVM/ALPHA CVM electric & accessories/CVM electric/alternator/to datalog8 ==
  Var : Inport
  Constant : Constant  Value=VerboseSignal
  Constant1 : Constant  Value=VerboseLevel
  Relational Operator : RelationalOperator  OutDataTypeStr=boolean  ZeroCross=off
  Subsystem : Subsystem
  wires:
  Constant1/1 -> Relational Operator/2
  Constant/1 -> Relational Operator/1
  Relational Operator/1 -> Subsystem/Enable
  Var/1 -> Subsystem/1(In1)

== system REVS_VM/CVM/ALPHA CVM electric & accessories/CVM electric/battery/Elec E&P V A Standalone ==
  volts_V : Inport
  curr_A : Inport  Port=2
  Compare To Constant : simulink/Logic and Bit Operations/Compare To Constant  relop=>=  const=1  OutDataTypeStr=boolean
  Constant : Constant  Value=VerboseSignal
  Subsystem : Subsystem
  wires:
  Constant/1 -> Compare To Constant/1
  Compare To Constant/1 -> Subsystem/Enable
  curr_A/1 -> Subsystem/2(curr_A)
  volts_V/1 -> Subsystem/1(volts_V)

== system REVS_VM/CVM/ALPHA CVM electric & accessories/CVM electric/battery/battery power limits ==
  note: Battery pack min and max voltage limited power limits seem to be too constrained compared with actual pack capacity so either the calculated limits are too low or the source data is overly conservative... so they are disabled for now until further investigation
  batt_temp_degC : Inport
  SoC_norm : Inport  Port=2
  OCV_V : Inport  Port=3
  volts_out_V : Inport  Port=4
  dis_res_Ohms : Inport  Port=5
  chg_res_Ohms : Inport  Port=6
  Bus Creator : BusCreator  Inputs=2
  Constant6 : Constant  Commented=on  Value=battery.min_voltage_V
  Constant7 : Constant  Commented=on  Value=battery.max_voltage_V
  Divide : Product  Commented=on  Inputs=**/
  Divide1 : Product  Commented=on  Inputs=**/
  Gain : Gain  Gain=-1
  MinMax : MinMax  Commented=on  Inputs=2
  MinMax1 : MinMax  Commented=on  Function=max  Inputs=2
  MinMax2 : MinMax  Commented=on  Inputs=2
  MinMax3 : MinMax  Commented=on  Inputs=2
  Product1 : Product  Inputs=3
  Product2 : Product  Inputs=3
  Sum : Sum  Commented=on  Inputs=+-
  Sum1 : Sum  Commented=on  Inputs=+-
  Sum2 : Sum  Commented=on  Inputs=-+
  Sum3 : Sum  Commented=on  Inputs=-+
  charge power limit : Subsystem
  charge temp derate : Lookup_n-D  NumberOfTableDimensions=1  BreakpointsForDimension1=battery.temperature_power_derate_index_temp_degC  IndexSearchMethod=Linear search  BeginIndexSearchUsingPreviousIndexResult=on  Table=battery.temperature_power_charge_derate_norm  ExtrapMethod=Clip  RndMeth=Simplest
  discharge  temp derate : Lookup_n-D  NumberOfTableDimensions=1  BreakpointsForDimension1=battery.temperature_power_derate_index_temp_degC  IndexSearchMethod=Linear search  BeginIndexSearchUsingPreviousIndexResult=on  Table=battery.temperature_power_discharge_derate_norm  ExtrapMethod=Clip  RndMeth=Simplest
  discharge power limit : Subsystem
  max SOC derate : Lookup_n-D  NumberOfTableDimensions=1  BreakpointsForDimension1=battery.charge_derate_soc_norm  IndexSearchMethod=Linear search  BeginIndexSearchUsingPreviousIndexResult=on  Table=[1 0]  ExtrapMethod=Clip  RndMeth=Simplest
  min SOC derate : Lookup_n-D  NumberOfTableDimensions=1  BreakpointsForDimension1=battery.discharge_derate_soc_norm  IndexSearchMethod=Linear search  BeginIndexSearchUsingPreviousIndexResult=on  Table=[0 1]  ExtrapMethod=Clip  RndMeth=Simplest
  max_dis_pwr_W : Outport
  max_chg_pwr_W : Outport  Port=2
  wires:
  Divide1/1 -> MinMax1/2
  Divide/1 -> MinMax/2
  Product1/1 -> max_dis_pwr_W/1, MinMax/1  "ees_max_discharge_power"
  charge temp derate/1 -> Product2/1
  Product2/1 -> MinMax1/1, max_chg_pwr_W/1  "ees_max_charge_power"
  min SOC derate/1 -> Product1/2
  Sum/1 -> Divide/1, Sum3/1
  max SOC derate/1 -> Product2/2
  charge power limit/1(out) -> Gain/1
  discharge power limit/1(out) -> Product1/3
  discharge  temp derate/1 -> Product1/1
  Constant7/1 -> Sum2/2, Sum1/2
  Sum1/1 -> Divide1/1, Sum2/1
  chg_res_Ohms/1 -> Divide1/3
  dis_res_Ohms/1 -> Divide/3
  Constant6/1 -> Sum3/2, Sum/2
  Gain/1 -> Product2/3
  OCV_V/1 -> MinMax2/1, MinMax3/2
  MinMax3/1 -> Sum1/1
  MinMax2/1 -> Sum/1
  volts_out_V/1 -> MinMax2/2, MinMax3/1
  Sum2/1 -> Divide1/2
  Sum3/1 -> Divide/2
  batt_temp_degC/1 -> Bus Creator/1, discharge  temp derate/1, charge temp derate/1  "temp_degC"
  Bus Creator/1 -> charge power limit/1(bus), discharge power limit/1(bus)
  SoC_norm/1 -> max SOC derate/1, min SOC derate/1, Bus Creator/2  "soc_norm"

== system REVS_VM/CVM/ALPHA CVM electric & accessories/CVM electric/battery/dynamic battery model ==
  batt_temp_degC : Inport
  curr_out_A : Inport  Port=2
  SOC : Subsystem
  dynamic voltage / loss model : Subsystem
  SoC_norm : Outport
  OCV_V : Outport  Port=2
  volts_out_V : Outport  Port=3
  dis_res_Ohm : Outport  Port=4
  chg_res_Ohm : Outport  Port=5
  loss_pwr_W : Outport  Port=6
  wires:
  dynamic voltage / loss model/5(loss_pwr_W) -> loss_pwr_W/1
  batt_temp_degC/1 -> SOC/2(batt_temp_degC), dynamic voltage / loss model/3(batt_temp_degC)
  SOC/2(chg_eff_norm) -> dynamic voltage / loss model/4(chg_eff_norm)
  dynamic voltage / loss model/1(OCV_V) -> OCV_V/1
  dynamic voltage / loss model/2(batt_volts_V) -> volts_out_V/1
  SOC/1(SoC_norm) -> dynamic voltage / loss model/2(SoC_norm), SoC_norm/1
  dynamic voltage / loss model/3(dis_res_Ohm) -> dis_res_Ohm/1
  dynamic voltage / loss model/4(chg_res_Ohm) -> chg_res_Ohm/1
  curr_out_A/1 -> dynamic voltage / loss model/1(batt_curr_A), SOC/1(batt_curr_A)
  SOC/3(pile_curr_A) -> dynamic voltage / loss model/5(pile_curr_A)

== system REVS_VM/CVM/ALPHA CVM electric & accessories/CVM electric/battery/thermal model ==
  loss_pwr_W : Inport
  amb_temp_degC : Inport  Port=2
  Constant1 : Constant  Value=battery.thermal.pack_heat_capacity_JpK
  Constant2 : Constant  Value=battery.thermal.initial_temp_degC
  Constant8 : Constant  Value=battery.thermal.pack_total_conductance_WpK
  Integrator1 : Integrator  InitialConditionSource=external
  Product : Product
  Product5 : Product  Inputs=*/
  Saturation : Saturate  UpperLimit=Inf  LowerLimit=eps
  Subtract : Sum  Inputs=|-+
  Sum3 : Sum  Inputs=|+-
  lowpass filter : TransferFcn  Denominator=[1 1]
  batt_temp_degC : Outport
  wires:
  Constant2/1 -> Integrator1/2
  Constant8/1 -> Product/1
  Constant1/1 -> Saturation/1
  amb_temp_degC/1 -> Subtract/1
  Subtract/1 -> Product/2
  Saturation/1 -> Product5/2
  Product/1 -> Sum3/2
  Integrator1/1 -> batt_temp_degC/1, Subtract/2
  Sum3/1 -> Product5/1
  Product5/1 -> Integrator1/1
  loss_pwr_W/1 -> lowpass filter/1
  lowpass filter/1 -> Sum3/1

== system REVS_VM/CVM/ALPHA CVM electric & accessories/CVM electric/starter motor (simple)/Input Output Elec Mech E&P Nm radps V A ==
  volts_in_V : Inport
  curr_in_A : Inport  Port=2
  trq_out_Nm : Inport  Port=3
  spd_out_radps : Inport  Port=4
  iner_out_kgm2 : Inport  Port=5
  Compare To Constant : simulink/Logic and Bit Operations/Compare To Constant  relop=>=  const=1  OutDataTypeStr=boolean
  Constant : Constant  Value=VerboseSignal
  Subsystem : Subsystem
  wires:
  volts_in_V/1 -> Subsystem/1(volts_in_V)
  curr_in_A/1 -> Subsystem/2(curr_in_A)
  trq_out_Nm/1 -> Subsystem/3(trq_out_Nm)
  spd_out_radps/1 -> Subsystem/4(spd_out_radps)
  iner_out_kgm2/1 -> Subsystem/5(iner_out_kgm2)
  Compare To Constant/1 -> Subsystem/Enable
  Constant/1 -> Compare To Constant/1

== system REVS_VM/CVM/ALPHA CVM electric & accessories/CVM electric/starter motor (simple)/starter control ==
  eng_on : Inport
  batt_volts_V : Inport  Port=2
  spd_in_radps : Inport  Port=3
  ISC_state : Inport  Port=4
  Compare To Constant : simulink/Logic and Bit Operations/Compare To Constant  relop=>=  const=1  OutDataTypeStr=boolean
  Compare To Constant1 : simulink/Logic and Bit Operations/Compare To Constant  relop=~=  const=0  OutDataTypeStr=boolean
  Compare To Zero : simulink/Logic and Bit Operations/Compare To Zero  relop===  OutDataTypeStr=boolean
  Gain : Gain  Gain=1.33
  Logical Operator : Logic  Operator=OR  AllPortsSameDT=off  OutDataTypeStr=boolean
  Logical Operator1 : Logic  AllPortsSameDT=off  OutDataTypeStr=boolean
  Logical Operator2 : Logic  AllPortsSameDT=off  OutDataTypeStr=boolean
  Relational Operator1 : RelationalOperator  OutDataTypeStr=boolean
  Relational Operator2 : RelationalOperator  Operator=<=  OutDataTypeStr=boolean
  boolean integrator : Subsystem
  cranking_speed_radps : Constant  Value=starter.cranking_speed_radps
  min volts : Constant  Value=starter.min_voltage_V
  starter state : Subsystem
  state : Outport
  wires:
  Compare To Constant/1 -> Logical Operator/1
  boolean integrator/1(out) -> Compare To Constant/1
  eng_on/1 -> Logical Operator1/1
  Logical Operator1/1 -> starter state/1(On)
  cranking_speed_radps/1 -> Gain/1
  batt_volts_V/1 -> Relational Operator2/1
  spd_in_radps/1 -> Relational Operator1/1, Compare To Zero/1
  Gain/1 -> Relational Operator1/2
  Relational Operator1/1 -> Logical Operator/2
  starter state/1(State) -> state/1
  Compare To Zero/1 -> Logical Operator1/2
  Relational Operator2/1 -> boolean integrator/1(bool)
  min volts/1 -> Relational Operator2/2
  Logical Operator/1 -> Logical Operator2/1
  Logical Operator2/1 -> starter state/2(Off)
  Compare To Constant1/1 -> Logical Operator2/2
  ISC_state/1 -> Compare To Constant1/1

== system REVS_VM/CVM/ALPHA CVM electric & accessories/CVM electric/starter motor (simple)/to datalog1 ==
  Var : Inport
  Constant : Constant  Value=VerboseSignal
  Constant1 : Constant  Value=VerboseLevel
  Relational Operator : RelationalOperator  OutDataTypeStr=boolean  ZeroCross=off
  Subsystem : Subsystem
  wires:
  Constant1/1 -> Relational Operator/2
  Constant/1 -> Relational Operator/1
  Relational Operator/1 -> Subsystem/Enable
  Var/1 -> Subsystem/1(In1)

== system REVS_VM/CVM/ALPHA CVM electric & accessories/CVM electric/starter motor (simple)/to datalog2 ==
  Var : Inport
  Constant : Constant  Value=VerboseSignal
  Constant1 : Constant  Value=VerboseLevel
  Relational Operator : RelationalOperator  OutDataTypeStr=boolean  ZeroCross=off
  Subsystem : Subsystem
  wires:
  Constant1/1 -> Relational Operator/2
  Constant/1 -> Relational Operator/1
  Relational Operator/1 -> Subsystem/Enable
  Var/1 -> Subsystem/1(In1)

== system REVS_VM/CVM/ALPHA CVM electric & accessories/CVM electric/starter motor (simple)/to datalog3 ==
  Var : Inport
  Constant : Constant  Value=VerboseSignal
  Constant1 : Constant  Value=VerboseLevel
  Relational Operator : RelationalOperator  OutDataTypeStr=boolean  ZeroCross=off
  Subsystem : Subsystem
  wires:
  Constant1/1 -> Relational Operator/2
  Constant/1 -> Relational Operator/1
  Relational Operator/1 -> Subsystem/Enable
  Var/1 -> Subsystem/1(In1)

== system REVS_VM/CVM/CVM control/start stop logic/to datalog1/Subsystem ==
  In1 : Inport
  Enable : EnablePort
  To Workspace : ToWorkspace  VariableName=datalog__controls__accel_anticipate_bool  SampleTime=-1
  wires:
  In1/1 -> To Workspace/1

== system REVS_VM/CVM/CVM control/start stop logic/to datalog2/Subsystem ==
  In1 : Inport
  Enable : EnablePort
  To Workspace : ToWorkspace  VariableName=datalog__controls__engine_on  SampleTime=-1
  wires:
  In1/1 -> To Workspace/1

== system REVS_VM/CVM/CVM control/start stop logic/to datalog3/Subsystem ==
  In1 : Inport
  Enable : EnablePort
  To Workspace : ToWorkspace  VariableName=datalog__controls__vehicle_stopped_bool  SampleTime=-1
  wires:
  In1/1 -> To Workspace/1

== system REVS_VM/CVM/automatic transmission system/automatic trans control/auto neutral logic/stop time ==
  bool : Inport
  Constant : Constant  Value=Normalize
  Data Type Conversion2 : DataTypeConversion  OutDataTypeStr=double
  Integrator1 : Integrator  ExternalReset=falling  LimitOutput=on  UpperSaturationLimit=UpperSaturationLimit  LowerSaturationLimit=0
  Switch : Switch  Criteria=u2 > Threshold
  normalize : Gain  Gain=1/UpperSaturationLimit
  out : Outport
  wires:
  Switch/1 -> out/1
  normalize/1 -> Switch/1
  Integrator1/1 -> Switch/3, normalize/1
  Constant/1 -> Switch/2
  bool/1 -> Data Type Conversion2/1
  Data Type Conversion2/1 -> Integrator1/1, Integrator1/2

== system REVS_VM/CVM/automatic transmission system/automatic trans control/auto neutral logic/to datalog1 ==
  Var : Inport
  Constant : Constant  Value=VerboseSignal
  Constant1 : Constant  Value=VerboseLevel
  Relational Operator : RelationalOperator  OutDataTypeStr=boolean  ZeroCross=off
  Subsystem : Subsystem
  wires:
  Constant1/1 -> Relational Operator/2
  Constant/1 -> Relational Operator/1
  Relational Operator/1 -> Subsystem/Enable
  Var/1 -> Subsystem/1(In1)
